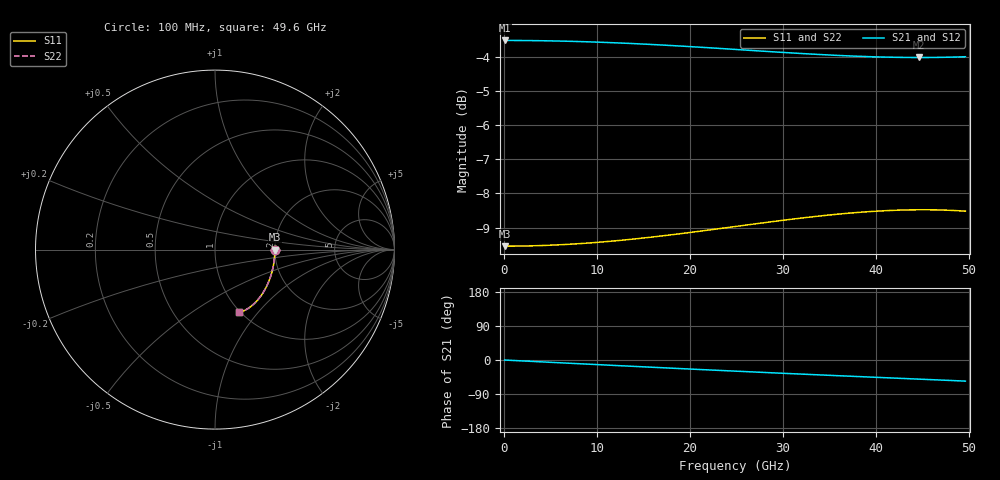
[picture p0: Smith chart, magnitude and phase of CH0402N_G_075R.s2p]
# GHz S RI R 75
! S-Parameters data
! Freq  reS11  imS11  reS21  imS21  reS12  imS12  reS22  imS22
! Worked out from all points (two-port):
!   100 points, 100 MHz to 49.6 GHz, reference 75 ohm
!   highest |S21| = -3.52 dB at 100 MHz (marker M1); lowest = -4.0 dB at 44.6 GHz (marker M2)
!   |S21| within 3 dB of the highest: start of sweep to end of sweep
!   lowest |S11| = -9.5 dB at 100 MHz (marker M3), VSWR 2.00, Z = 150 - j0.319 ohm
!   |S11| at or under -10 dB: nowhere
!   |S22| runs from -9.5 to -8.5 dB; largest |S21 - S12| = 0
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0.1  0.3333 -0.000946  0.6667 -0.00141  0.6667 -0.00141  0.3333 -0.000946
2.1  0.3329 -0.0199  0.6658 -0.0296  0.6658 -0.0296  0.3329 -0.0199
4.1  0.3318 -0.0387  0.6635 -0.0577  0.6635 -0.0577  0.3318 -0.0387
6.1  0.33 -0.0575  0.6598 -0.0855  0.6598 -0.0855  0.33 -0.0575
8.6  0.3267 -0.0808  0.653 -0.1197  0.653 -0.1197  0.3267 -0.0808
10.6  0.3232 -0.0993  0.6461 -0.1466  0.6461 -0.1466  0.3232 -0.0993
12.6  0.319 -0.1176  0.6378 -0.1729  0.6378 -0.1729  0.319 -0.1176
14.6  0.3142 -0.1356  0.6284 -0.1986  0.6284 -0.1986  0.3142 -0.1356
16.6  0.3086 -0.1533  0.6177 -0.2235  0.6177 -0.2235  0.3086 -0.1533
18.6  0.3023 -0.1706  0.6061 -0.2475  0.6061 -0.2475  0.3023 -0.1706
21.1  0.2935 -0.1918  0.5901 -0.2764  0.5901 -0.2764  0.2935 -0.1918
23.1  0.2857 -0.2082  0.5764 -0.2985  0.5764 -0.2985  0.2857 -0.2082
25.1  0.2772 -0.2241  0.562 -0.3197  0.562 -0.3197  0.2772 -0.2241
29.1  0.2584 -0.2541  0.5313 -0.3594  0.5313 -0.3594  0.2584 -0.2541
33.1  0.2371 -0.2813  0.4989 -0.3956  0.4989 -0.3956  0.2371 -0.2813
35.6  0.2228 -0.2966  0.478 -0.4167  0.478 -0.4167  0.2228 -0.2966
37.6  0.2108 -0.3077  0.4611 -0.4329  0.4611 -0.4329  0.2108 -0.3077
39.6  0.1985 -0.3178  0.444 -0.4484  0.444 -0.4484  0.1985 -0.3178
41.6  0.1859 -0.3268  0.4268 -0.4635  0.4268 -0.4635  0.1859 -0.3268
44.6  0.1667 -0.3379  0.4006 -0.4856  0.4006 -0.4856  0.1667 -0.3379
47.1  0.1508 -0.345  0.3784 -0.5035  0.3784 -0.5035  0.1508 -0.345
49.6  0.1353 -0.3498  0.3556 -0.5214  0.3556 -0.5214  0.1353 -0.3498
